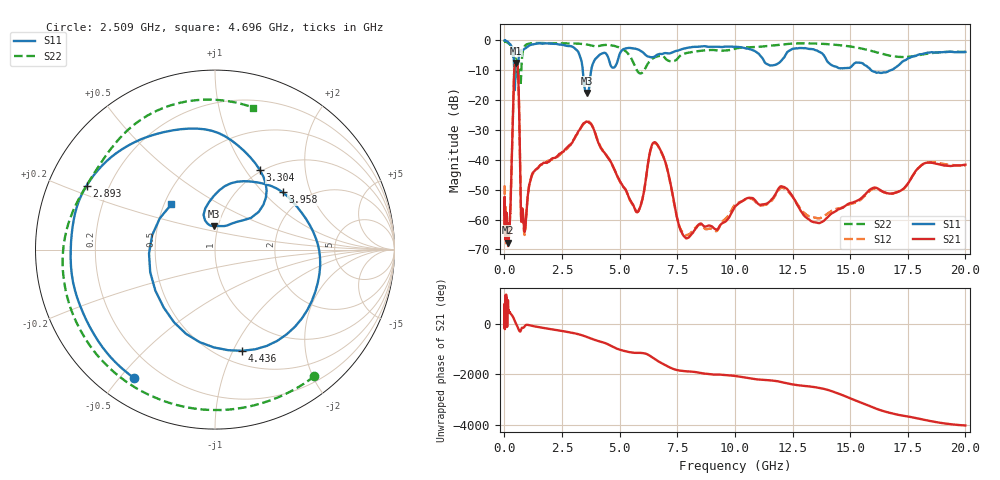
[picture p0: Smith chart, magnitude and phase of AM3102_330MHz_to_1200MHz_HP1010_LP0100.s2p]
! Date/Time: Tue, Sep 11, 2018 5:19 PM
! Network Analyzer: Agilent Technologies E8362B Rev: A.07.50.63
! Sweep from 0.010 to 20.000 GHz, 1601 Points, Sweep Type: LOG
! Power Supply: 4.949 V, 0.001 A
# Hz S DB R 50
!freq MagS11 AngS11 MagS21 AngS21 MagS12 AngS12 MagS22 AngS22
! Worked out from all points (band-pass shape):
!   1601 points, 10 MHz to 20 GHz, reference 50 ohm
!   highest |S21| = -7.53 dB at 484.8 MHz (marker M1); lowest = -67.7 dB at 167.3 MHz (marker M2)
!   |S21| within 3 dB of the highest: 424.9 MHz to 592.3 MHz (167.4 MHz wide, 32.9 % of centre)
!   lowest |S11| = -17.6 dB at 3.599 GHz (marker M3), VSWR 1.30, Z = 47.7 + j12.8 ohm
!   |S11| at or under -10 dB: 425.3 MHz to 478.2 MHz (52.98 MHz wide, 11.7 % of centre); 3.402 GHz to 3.767 GHz (365 MHz wide, 10.2 % of centre); 15.91 GHz to 16.76 GHz (845.7 MHz wide, 5.18 % of centre)
!   |S22| runs from -15.1 to -0.2 dB; largest |S21 - S12| = 0.0058
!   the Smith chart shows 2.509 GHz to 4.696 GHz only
!   S11 on the Smith chart (normalised r, x): 2.509 GHz: 0.11, -0.55; 2.893 GHz: 0.12, +0.23; 3.304 GHz: 0.97, +1.17; 3.958 GHz: 1.54, +1.30; 4.436 GHz: 0.64, -1.09; 4.696 GHz: 0.55, +0.31
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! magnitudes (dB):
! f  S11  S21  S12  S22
! 10 MHz  0.0  -53.2  -48.9  -0.2
! 35.55 MHz  0.0  -65.8  -63.5  -0.3
! 126.4 MHz  -0.4  -66.1  -65.8  -0.7
! 167.3 MHz  -0.6  -67.7  -68.0  -0.9
! 263.9 MHz  -1.4  -56.1  -56.3  -1.7
! 447.2 MHz  -16.6  -8.2  -8.3  -6.5
! 484.8 MHz  -8.9  -7.5  -7.6  -6.1
! 594.7 MHz  -7.6  -10.9  -11.0  -12.8
! 722.6 MHz  -3.3  -59.3  -58.5  -12.4
! 865.5 MHz  -2.8  -63.6  -64.5  -2.1
! 1.59 GHz  -1.0  -41.6  -41.6  -0.9
! 2.509 GHz  -1.5  -37.4  -37.6  -0.9
! 2.893 GHz  -1.9  -34.7  -34.5  -1.0
! 3.304 GHz  -5.9  -29.4  -29.4  -1.1
! 3.599 GHz  -17.6  -27.2  -27.1  -1.4
! 3.958 GHz  -6.1  -31.6  -31.5  -2.0
! 4.436 GHz  -4.7  -38.7  -38.5  -1.5
! 4.696 GHz  -9.1  -42.0  -42.0  -1.7
! 5.652 GHz  -2.7  -56.3  -56.3  -8.4
! 6.549 GHz  -5.3  -34.1  -34.4  -5.6
! 7.92 GHz  -2.5  -66.3  -65.2  -4.2
! 20 GHz  -3.9  -41.6  -42.0  -3.8
